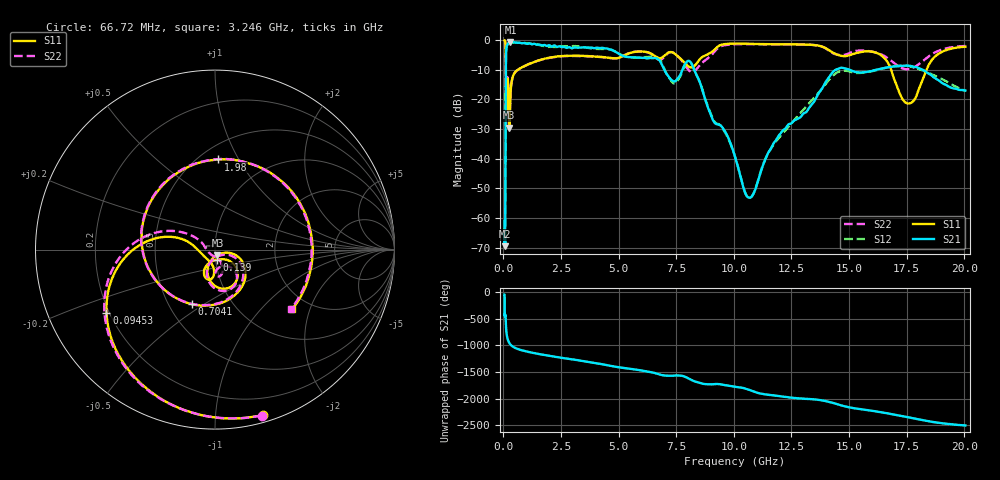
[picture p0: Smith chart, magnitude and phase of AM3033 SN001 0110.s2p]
# Hz S DB R 50
!freq MagS11 AngS11 MagS21 AngS21 MagS12 AngS12 MagS22 AngS22
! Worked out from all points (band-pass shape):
!   1601 points, 50 MHz to 20.05 GHz, reference 50 ohm
!   highest |S21| = -0.71 dB at 300.8 MHz (marker M1); lowest = -69.5 dB at 70.84 MHz (marker M2)
!   |S21| within 3 dB of the highest: 118.6 MHz to 4.797 GHz (4.678 GHz wide, 190 % of centre)
!   lowest |S11| = -29.5 dB at 255.1 MHz (marker M3), VSWR 1.07, Z = 51.3 - j3.15 ohm
!   |S11| at or under -10 dB: 101.4 MHz to 627.9 MHz (526.5 MHz wide, 144 % of centre); 16.83 GHz to 18.36 GHz (1.539 GHz wide, 8.75 % of centre)
!   |S22| runs from -29.1 to -0.1 dB; largest |S21 - S12| = 0.063
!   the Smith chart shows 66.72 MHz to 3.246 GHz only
!   S11 on the Smith chart (normalised r, x): 66.72 MHz: 0.06, -1.33; 94.53 MHz: 0.19, -0.26; 139 MHz: 1.01, -0.12; 704.1 MHz: 0.65, -0.45; 1.98 GHz: 0.61, +0.83; 3.246 GHz: 1.62, -1.53
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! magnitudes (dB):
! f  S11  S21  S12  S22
! 50 MHz  -0.1  -60.9  -69.0  -0.1
! 66.72 MHz  -0.4  -66.5  -66.4  -0.4
! 70.84 MHz  -0.4  -69.5  -67.5  -0.4
! 94.53 MHz  -3.1  -25.2  -25.2  -3.2
! 109.4 MHz  -23.0  -5.7  -5.7  -28.9
! 135.9 MHz  -23.4  -2.3  -2.3  -19.7
! 139 MHz  -24.8  -2.2  -2.2  -19.9
! 183.5 MHz  -13.0  -1.4  -1.4  -12.7
! 255.1 MHz  -29.5  -0.8  -0.8  -27.6
! 300.8 MHz  -18.6  -0.7  -0.7  -18.9
! 369.6 MHz  -13.4  -0.8  -0.8  -13.6
! 704.1 MHz  -9.6  -0.9  -1.0  -9.6
! 1.005 GHz  -8.5  -1.3  -1.1  -8.4
! 1.98 GHz  -6.0  -1.7  -2.3  -6.0
! 2.722 GHz  -5.3  -2.6  -2.2  -5.4
! 3.246 GHz  -5.3  -2.6  -2.1  -5.4
! 7.402 GHz  -4.4  -14.0  -14.6  -4.4
! 8.251 GHz  -9.0  -9.4  -9.5  -10.8
! 10.69 GHz  -1.3  -53.1  -53.2  -1.4
! 14.53 GHz  -5.0  -9.7  -10.8  -5.0
! 17.59 GHz  -21.4  -8.7  -8.8  -9.8
! 20.05 GHz  -2.2  -17.1  -17.1  -2.0
